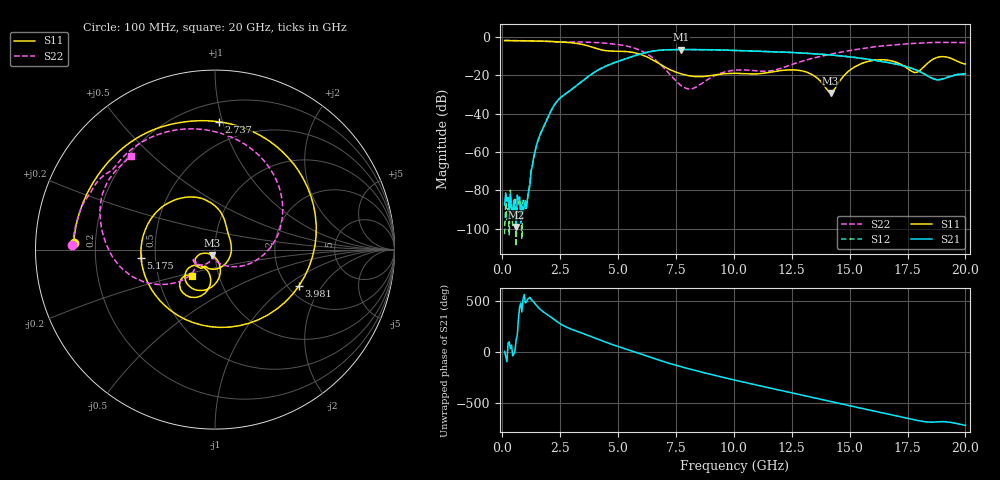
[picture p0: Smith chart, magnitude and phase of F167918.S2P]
!  2-Port S-parameters saved by WinCal
! VAR MeasName=S-Parameters (CALIBRATED_DATA) read from VNA (N5242A)
! VAR MeasDate=2016-11-22 10:24:43
! VAR NAME=F167918
! VAR FILENAME=F167918.S2P
! VAR DATE=2016-11-22 10:24:43
! VAR PHYS_PORTS=1,2
# Hz S DB R 50
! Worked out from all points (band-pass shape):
!   401 points, 100 MHz to 20 GHz, reference 50 ohm
!   highest |S21| = -6.71 dB at 7.712 GHz (marker M1); lowest = -99.0 dB at 597.5 MHz (marker M2)
!   |S21| within 3 dB of the highest: 5.769 GHz to 14.32 GHz (8.547 GHz wide, 85.1 % of centre)
!   lowest |S11| = -29.3 dB at 14.18 GHz (marker M3), VSWR 1.07, Z = 48.1 - j2.82 ohm
!   |S11| at or under -10 dB: 6.141 GHz to end of sweep
!   |S22| runs from -27.3 to -2.0 dB; largest |S21 - S12| = 0.0049
!   S11 on the Smith chart (normalised r, x): 100 MHz: 0.12, +0.02; 2.737 GHz: 0.34, +0.97; 3.981 GHz: 2.29, -1.25; 5.175 GHz: 0.42, -0.05; 20 GHz: 0.75, -0.23
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1e8  -2.07 177.3  -87.63 4.9  -102.77 7.2  -2.00 178.3
5.975e8  -2.13 164.0  -98.98 115.2  -108.99 27.0  -2.07 170.3
1.095e9  -2.22 150.4  -83.42 157.7  -85.37 179.9  -2.16 162.2
1.64225e9  -2.33 133.7  -50.77 57.2  -50.57 55.7  -2.37 153.7
2.73675e9  -2.95 88.3  -29.72 -113.3  -29.73 -113.7  -2.79 136.9
3.43325e9  -4.01 38.7  -23.36 -175.6  -23.39 -175.7  -2.81 123.0
3.9805e9  -5.85 -23.3  -18.53 137.1  -18.52 137.2  -3.05 109.6
4.478e9  -7.32 -93.1  -15.34 93.4  -15.29 93.4  -3.46 95.4
5.1745e9  -7.65 -173.5  -12.17 39.0  -12.13 38.5  -4.47 70.5
5.92075e9  -9.09 126.9  -9.17 -16.4  -9.19 -16.9  -6.94 33.1
6.7665e9  -14.01 78.6  -7.13 -81.1  -7.17 -81.3  -13.78 -23.1
7.71175e9  -19.35 43.7  -6.71 -145.9  -6.73 -145.8  -25.40 -93.6
8.657e9  -20.73 -23.2  -6.76 157.5  -6.77 157.5  -24.07 -110.8
1.005e10  -19.11 -105.3  -7.19 81.2  -7.19 81.3  -17.46 -146.1
1.1642e10  -18.44 -123.6  -7.81 0.0  -7.79 -0.0  -17.67 -144.6
1.338325e10  -19.84 -160.3  -8.83 -88.0  -8.83 -87.8  -11.32 -138.6
1.417925e10  -29.27 -121.6  -9.53 -128.3  -9.54 -128.0  -9.14 -146.4
1.53235e10  -15.06 -85.8  -11.00 173.7  -10.96 174.1  -6.57 -159.9
1.67165e10  -12.41 -132.6  -13.61 104.8  -13.58 104.9  -4.51 179.5
1.7811e10  -18.70 -125.4  -17.08 50.3  -16.98 50.4  -3.51 163.4
1.89055e10  -10.49 -118.0  -22.43 33.1  -22.22 32.7  -3.00 146.3
2e10  -14.18 -130.3  -19.42 -4.0  -19.27 -4.2  -3.10 132.2
